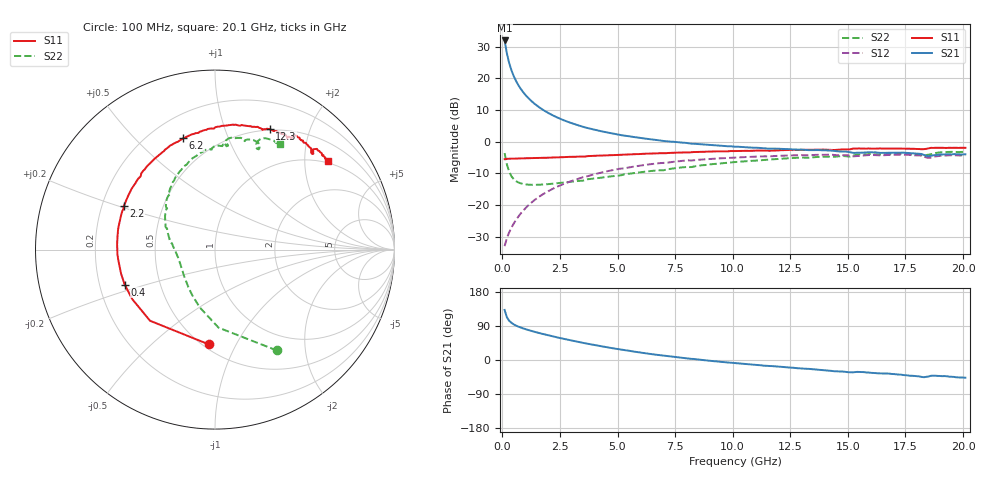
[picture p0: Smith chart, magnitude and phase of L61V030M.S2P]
!  Infineon Technologies AG
! BFR380L3 , PF131585-7, No.6, Th 09.10.01, soldered on pcb-board, measured with PP GSG850
!  Vce=1.0 V,  Ic=30.0 mA
! Common Emitter S-Parameters:  15. November 2001
#  GHz  S  MA  R  50
! f  S11  S21  S12  S22
! GHz  Mag  Ang  Mag  Ang  Mag  Ang  Mag  Ang
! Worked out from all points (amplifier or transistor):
!   201 points, 100 MHz to 20.1 GHz, reference 50 ohm
!   highest |S21| = 31.9 dB at 100 MHz (marker M1)
!   |S21| within 3 dB of that: start of sweep to 172.5 MHz
!   unconditionally stable (mu >= 1): 1.079 GHz to 4.72 GHz; 18.4 GHz to 18.5 GHz
!   at 3.4 GHz: K = 1.02, MAG = 7.3 dB, |S12| = -11.5 dB
!   at 10.1 GHz: K = 0.97, MSG = 1.7 dB, |S12| = -5.0 dB
!   at 20.1 GHz: K = 0.99, MSG = 0.2 dB, |S12| = -4.3 dB
!   S11 on the Smith chart (normalised r, x): 100 MHz: 0.53, -0.78; 400 MHz: 0.31, -0.17; 2.2 GHz: 0.29, +0.21; 6.2 GHz: 0.33, +0.70; 12.3 GHz: 0.49, +1.44; 20.1 GHz: 0.94, +2.58
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0.1  0.5288 -93.9  39.55 132.0  0.0224 57.2  0.6594 -58.5
0.2  0.5368 -132.4  24.55 112.4  0.0302 53.8  0.4352 -87.4
0.3  0.5374 -149.1  17.3 103.4  0.03712 56.3  0.3336 -104.6
0.4  0.5397 -158.8  13.26 97.8  0.0442 58.5  0.2828 -116.8
0.5  0.5402 -165.5  10.72 93.8  0.05117 61.2  0.2544 -126.1
0.6  0.5399 -170.1  9 90.7  0.05854 62.8  0.2373 -133.3
0.7  0.5423 -174.2  7.755 88.0  0.06587 64.1  0.2266 -139.3
0.8  0.5445 -177.6  6.81 85.6  0.07355 65.2  0.2195 -144.2
1  0.5463 177.0  5.487 81.5  0.08881 66.0  0.2117 -151.8
1.2  0.5481 172.4  4.599 77.8  0.1042 66.2  0.2088 -157.5
1.5  0.5524 166.3  3.713 72.7  0.1274 65.7  0.2083 -164.1
1.8  0.5558 161.2  3.121 68.1  0.1506 64.4  0.2108 -169.2
2.2  0.5625 154.5  2.59 62.3  0.1807 62.2  0.2171 -174.8
3.5  0.5815 136.0  1.716 45.2  0.2742 53.4  0.2422 171.5
4.8  0.6129 120.5  1.344 30.9  0.3555 43.9  0.2853 158.6
6.2  0.6449 106.0  1.118 18.0  0.4297 33.6  0.336 145.8
6.8  0.6552 100.4  1.049 12.9  0.4566 29.1  0.3527 140.0
10.1  0.7101 76.7  0.8329 -8.2  0.5608 7.7  0.4758 114.7
12.3  0.738 65.6  0.7635 -19.1  0.6043 -5.3  0.544 98.8
13.5  0.7435 60.0  0.7369 -24.5  0.6145 -11.9  0.5673 91.4
16.8  0.7769 47.8  0.6707 -36.0  0.6167 -26.9  0.6413 73.0
20.1  0.7992 38.3  0.632 -46.6  0.61 -40.0  0.6903 58.3
